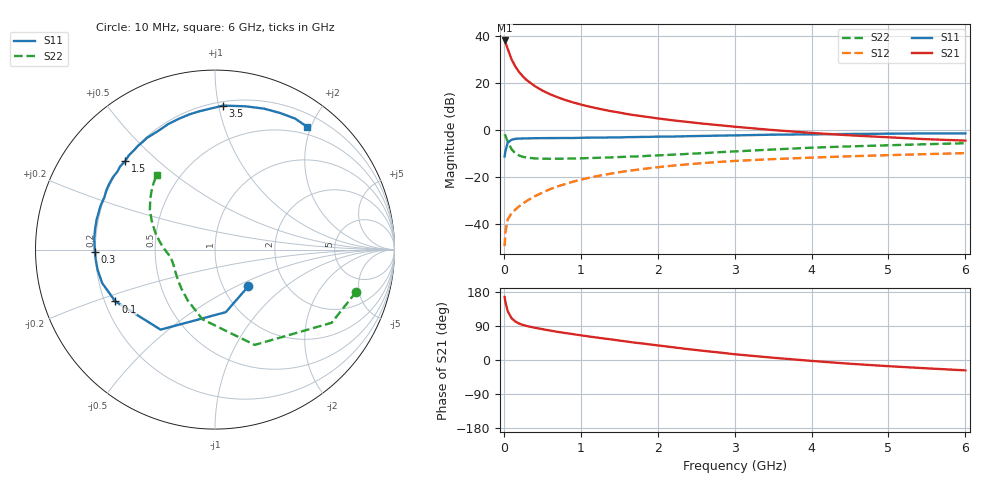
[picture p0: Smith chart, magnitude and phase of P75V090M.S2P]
! SIEMENS Small Signal Semiconductors
! BFP196
! Si NPN RF Bipolar Junction Transistor in SOT143
! VCE = 5 V  IC = 90 mA
! Common Emitter S-Parameters:  May  1996
# GHz  S  MA  R  50
!  f  S11  S21  S12  S22
! GHz  MAG  ANG  MAG  ANG  MAG  ANG  MAG  ANG
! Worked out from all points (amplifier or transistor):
!   36 points, 10 MHz to 6 GHz, reference 50 ohm
!   highest |S21| = 38.2 dB at 10 MHz (marker M1)
!   |S21| within 3 dB of that: start of sweep to 43.85 MHz
!   unconditionally stable (mu >= 1): 368.6 MHz to 4.571 GHz
!   at 250 MHz: K = 0.91, MSG = 27.0 dB, |S12| = -31.2 dB
!   at 1.4 GHz: K = 1.09, MAG = 11.4 dB, |S12| = -18.5 dB
!   at 6 GHz: K = 0.98, MSG = 2.7 dB, |S12| = -9.8 dB
!   S11 on the Smith chart (normalised r, x): 10 MHz: 1.31, -0.58; 100 MHz: 0.24, -0.23; 300 MHz: 0.20, -0.01; 1.5 GHz: 0.20, +0.39; 3.5 GHz: 0.23, +1.03; 6 GHz: 0.38, +1.94
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0.01  0.2764 -47.7  81.38 166.4  0.0034 79.7  0.8206 -16.7
0.02  0.3536 -80.2  74.69 153.7  0.0067 67.5  0.7672 -32.1
0.05  0.5392 -124.2  53.88 129.0  0.0126 53.7  0.5752 -67.4
0.1  0.6257 -152.5  32.41 110.2  0.017 50.3  0.3945 -100.2
0.15  0.6559 -163.5  22.57 101.4  0.0204 52.0  0.3212 -118.2
0.2  0.6641 -170.5  17.23 96.0  0.0241 56.4  0.2885 -130.0
0.25  0.6668 -175.3  13.81 92.4  0.0276 58.0  0.2703 -138.8
0.3  0.6696 -179.0  11.57 89.6  0.0314 61.6  0.2609 -144.3
0.4  0.6756 174.9  8.743 85.2  0.0392 63.6  0.2513 -152.8
0.5  0.6777 170.4  6.994 81.5  0.0467 64.8  0.2471 -158.1
0.6  0.6801 166.0  5.837 77.7  0.0555 65.4  0.2465 -161.8
0.7  0.6808 161.9  5.012 74.2  0.0637 64.9  0.2469 -164.4
0.8  0.6828 159.0  4.388 71.2  0.0716 64.1  0.2485 -166.7
1.1  0.6938 148.3  3.211 62.3  0.0962 61.5  0.2553 -171.7
1.5  0.702 135.5  2.382 51.4  0.1275 56.0  0.2683 -176.5
1.7  0.7144 129.0  2.085 45.8  0.1418 53.1  0.2762 -179.4
2.2  0.7326 115.8  1.621 33.6  0.1763 45.5  0.3011 174.3
2.8  0.7667 100.7  1.278 19.8  0.2112 36.4  0.3406 165.3
3.5  0.8036 86.8  1.007 6.0  0.2427 26.3  0.3887 155.3
4.5  0.8316 70.8  0.778 -9.9  0.2788 14.2  0.4528 142.9
5.5  0.8555 58.6  0.643 -22.0  0.31 3.5  0.5041 132.8
6  0.8554 53.1  0.601 -27.4  0.3248 -2.2  0.5284 127.9
